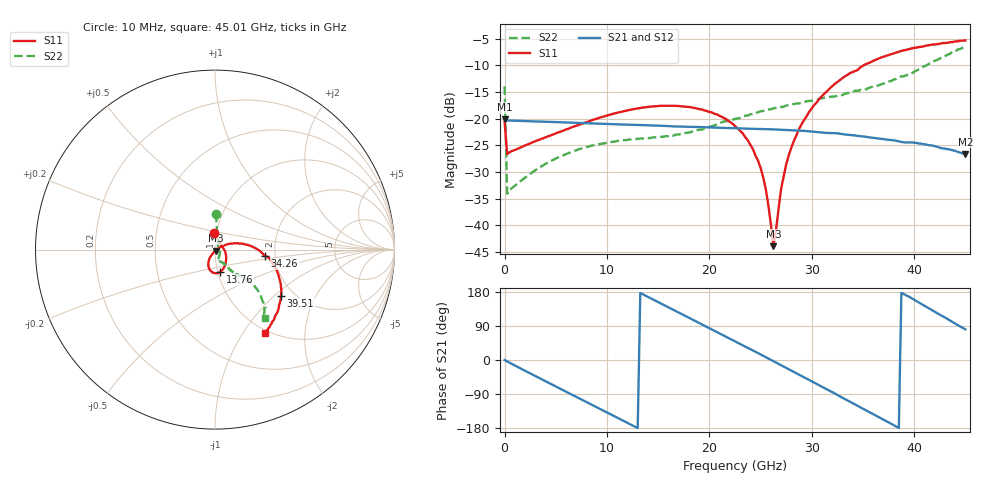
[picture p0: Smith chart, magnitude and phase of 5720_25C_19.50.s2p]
! Device:  ADRF5720
! Description: 0.5dB LSB GaAs MMIC 6-bit Digital Attenuator
! Frequency:  0.000009 -  40 GHz
! Ports:
!	RF1	= Port 1
!	RF2	= Port 2
! Vdd:  3.3 Volt
! Vss:  -3.3 Volt
! Control:  0/3.3 Volt
! State:  19.50 dB attenuation
! Data:  The device was measured using G-S-G Probes on a matrix board.
!  Data was collected using an calibrated 4 port network analyzer.
!  The reference plane for this measurement is at the launchers.
! Note:  Analog Devices supplies this data as a sample of measured data
!  for this product.  Your particular data for this product may vary.
!  Data was taken at 25 degrees C.
!  Analog Devices reserves the right to change this data at anytime.
# GHZ S DB R 45.0
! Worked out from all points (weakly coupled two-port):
!   181 points, 10 MHz to 45.01 GHz, reference 45 ohm
!   highest |S21| = -20.16 dB at 10 MHz (marker M1); lowest = -26.6 dB at 45.01 GHz (marker M2)
!   lowest |S11| = -43.9 dB at 26.26 GHz (marker M3), VSWR 1.01, Z = 45.3 - j0.488 ohm
!   |S11| at or under -10 dB: start of sweep to 35.08 GHz
!   |S22| runs from -34.1 to -6.5 dB; largest |S21 - S12| = 0.00015
!   S11 on the Smith chart (normalised r, x): 10 MHz: 0.97, +0.18; 13.76 GHz: 1.03, -0.26; 34.26 GHz: 1.76, -0.14; 39.51 GHz: 1.72, -1.10; 45.01 GHz: 0.96, -1.25
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0.01  -20.50 95.0  -20.16 -0.1  -20.16 -0.1  -13.93 88.6
0.26  -26.65 10.5  -20.35 -3.9  -20.35 -3.9  -34.06 24.4
3.51  -23.87 -20.7  -20.56 -49.2  -20.56 -49.2  -29.05 -40.9
7.76  -20.80 -48.0  -20.84 -107.6  -20.84 -107.6  -25.45 -69.5
13.76  -17.88 -76.9  -21.25 170.0  -21.25 170.0  -23.70 -76.0
15.26  -17.60 -83.5  -21.34 149.2  -21.34 149.2  -23.42 -73.7
19.26  -18.28 -101.2  -21.60 94.2  -21.60 94.2  -22.07 -62.4
22.76  -21.79 -117.1  -21.82 45.8  -21.82 45.9  -19.99 -55.6
24.01  -24.90 -121.9  -21.90 28.6  -21.91 28.6  -19.21 -54.7
25.01  -29.24 -122.2  -21.93 14.7  -21.93 14.7  -18.63 -54.2
25.51  -33.15 -116.9  -21.96 7.5  -21.96 7.5  -18.39 -54.5
26.26  -43.91 -57.6  -22.02 -3.0  -22.02 -3.0  -18.07 -52.7
26.51  -40.97 -9.5  -22.04 -6.5  -22.05 -6.5  -17.97 -54.2
27.01  -33.21 18.9  -22.07 -13.6  -22.07 -13.6  -17.83 -53.5
27.76  -26.89 26.2  -22.16 -24.2  -22.17 -24.2  -17.44 -53.1
28.76  -21.97 22.9  -22.25 -38.4  -22.25 -38.3  -17.15 -53.3
30.26  -17.43 15.3  -22.46 -60.0  -22.46 -59.9  -16.51 -52.4
32.26  -13.49 4.2  -22.72 -88.3  -22.72 -88.3  -15.85 -50.8
34.26  -11.07 -7.3  -23.16 -117.7  -23.16 -117.7  -14.76 -48.4
37.76  -7.90 -25.8  -24.01 -168.0  -24.01 -168.0  -12.96 -43.9
39.51  -6.97 -34.8  -24.47 167.0  -24.47 167.0  -11.82 -43.9
45.01  -5.35 -59.3  -26.65 80.8  -26.64 80.8  -6.54 -53.5
